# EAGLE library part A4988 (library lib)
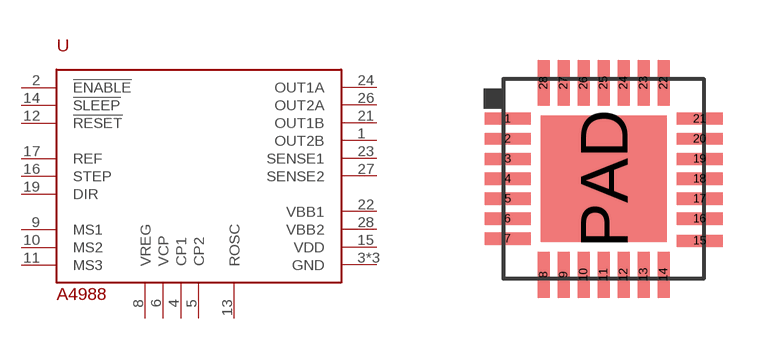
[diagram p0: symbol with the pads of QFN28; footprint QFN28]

Designator prefix -

## A4988  [QFN28]
1  OUT2B
2  !ENABLE
3  GND
4  CP1
5  CP2
6  VCP
8  VREG
9  MS1
10  MS2
11  MS3
12  !RESET
13  ROSC
14  !SLEEP
15  VDD
16  STEP
17  REF
18  GND
19  DIR
21  OUT1B
22  VBB1
23  SENSE1
24  OUT1A
26  OUT2A
27  SENSE2
28  VBB2
PAD  GND

## Footprint QFN28 (pad centres in mm)
smd 1.15 x 0.3: 1 -2.4,1.5; 2 -2.4,1; 3 -2.4,0.5; 4 -2.4,0; 5 -2.4,-0.5; 6 -2.4,-1; 7 -2.4,-1.5; 15 2.4,-1.55; 16 2.4,-1; 17 2.4,-0.5; 18 2.4,0; 19 2.4,0.5; 20 2.4,1; 21 2.4,1.5
smd 0.3 x 1.15: 8 -1.5,-2.4; 9 -1,-2.4; 10 -0.5,-2.4; 11 0,-2.4; 12 0.5,-2.4; 13 1,-2.4; 14 1.5,-2.4; 22 1.5,2.4; 23 1,2.4; 24 0.5,2.4; 25 0,2.4; 26 -0.5,2.4; 27 -1,2.4; 28 -1.5,2.4
smd 3.15 x 3.15: PAD 0,0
